{attribute 'qualified_only'}
VAR_GLOBAL PERSISTENT
	LID_HEATER_PID				:ARRAY[1..10] OF STR_PID;
	CHAMBER_HEATER_PID			:ARRAY[1..10] OF STR_PID;
	PEN_VALVE_HEATER_PID		:STR_PID;
	GATE_VALVE_HEATER_PID		:STR_PID;
	IGS_HEATER_PID				:ARRAY[1..10] OF STR_PID;
	TAPE_HEATER_PID				:ARRAY[1..10] OF STR_PID;
	FORELINE_HEATER_PID			:ARRAY[1..20] OF STR_PID;
	STAGE_HEATER_PID			:ARRAY[1..10] OF STR_PID;
END_VAR
